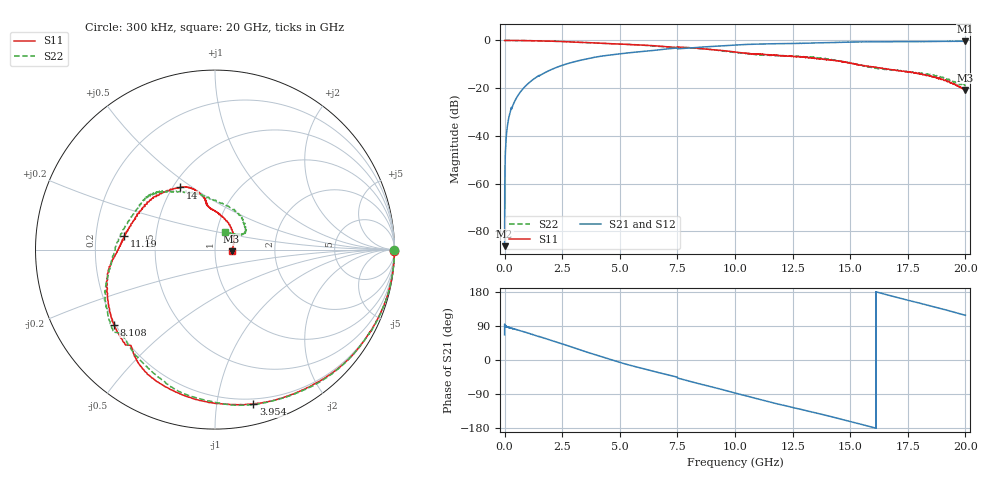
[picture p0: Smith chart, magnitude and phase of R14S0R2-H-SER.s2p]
!{R14S0R2}
!Johanson Technology Inc.
!www.johansontechnology.com
!Test Board Conditions:
!Substrate Type  RO4350B
!Substrate Thickness  20 mil
!Substrate Dk  3.66
!TL Type: GCPW
!TL Trace Width  36 mil
!TL Gap  12 mil
!Electrode orientation  Horizontal
!DUT TOPOLOGY	SERIES
!Mounting Pad LxW  26x36 mil
! Created Wed Nov 25 17:33:21 2020
! 2 Port Network Data from SP1.SP block
! freq  magS11  angS11  magS21  angS21  magS12  angS12  magS22  angS22
# khz S ma R 50
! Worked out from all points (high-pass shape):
!   20001 points, 300 kHz to 20 GHz, reference 50 ohm
!   highest |S21| = -0.32 dB at 20 GHz (marker M1); lowest = -86.2 dB at 300 kHz (marker M2)
!   |S21| within 3 dB of the highest: 7.324 GHz to 7.5 GHz (175.4 MHz wide, 2.37 % of centre); 7.801 GHz to end of sweep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
!   lowest |S11| = -20.7 dB at 20 GHz (marker M3), VSWR 1.20, Z = 60.1 - j1.1 ohm
!   |S11| at or under -10 dB: 15.25616 GHz to 15.25658 GHz (421.3 kHz wide, 0.00276 % of centre); 15.26 GHz to end of sweep
!   |S22| runs from -19.2 to 0.0 dB; largest |S21 - S12| = 0.016
!   S11 on the Smith chart (normalised r, x): 300 kHz: open; 3.954 GHz: 0.16, -1.27; 8.108 GHz: 0.19, -0.32; 11.19 GHz: 0.32, +0.06; 14 GHz: 0.55, +0.45; 20 GHz: 1.20, -0.02
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300  0.9954 -0.3  4.921e-05 66.4  3.641e-05 17.7  0.9969 -0.2
103300  0.9995 -2.0  0.01364 87.8  0.01376 87.5  0.9999 -2.1
146300  0.9994 -2.8  0.01947 86.9  0.01958 87.1  0.9998 -2.9
279300  0.9987 -5.6  0.03706 83.8  0.03723 83.9  0.999 -5.7
542300  0.9977 -9.9  0.06579 79.6  0.06603 79.7  0.9966 -10.0
903300  0.9929 -16.4  0.1105 73.2  0.1104 73.2  0.9923 -16.8
1399300  0.9812 -26.1  0.1727 63.6  0.1734 63.5  0.9824 -26.7
2447300  0.9501 -45.4  0.2952 43.5  0.2952 43.5  0.9497 -47.1
3334300  0.9114 -63.3  0.3894 25.7  0.3901 25.6  0.9105 -65.1
3954300  0.8867 -76.0  0.4484 13.4  0.4482 13.3  0.8867 -77.0
5488300  0.8188 -106.8  0.5578 -14.6  0.5567 -14.5  0.8224 -102.0
6667300  0.7632 -123.9  0.6342 -33.0  0.6363 -32.7  0.7532 -120.9
7600300  0.725 -134.8  0.674 -49.2  0.6786 -49.2  0.7226 -142.4
8108300  0.7013 -143.5  0.6988 -57.4  0.7044 -57.2  0.6935 -149.9
1.00003e7  0.5755 -174.2  0.8004 -87.1  0.8051 -87.1  0.5628 -178.9
1.11943e7  0.5119 171.7  0.8423 -105.8  0.8476 -106.3  0.494 156.3
1.33343e7  0.4286 132.1  0.8855 -137.3  0.8799 -137.3  0.4417 133.8
1.40003e7  0.3965 119.1  0.9004 -146.9  0.8973 -147.0  0.4085 128.1
1.53593e7  0.3115 103.6  0.93 -167.9  0.926 -167.8  0.3143 103.5
1.66673e7  0.2503 99.6  0.941 170.9  0.9453 171.6  0.2484 64.1
1.86943e7  0.1675 65.3  0.9539 139.3  0.9576 139.5  0.181 29.1
2e7  0.09244 -5.6  0.9642 118.0  0.9598 118.0  0.1103 61.3
